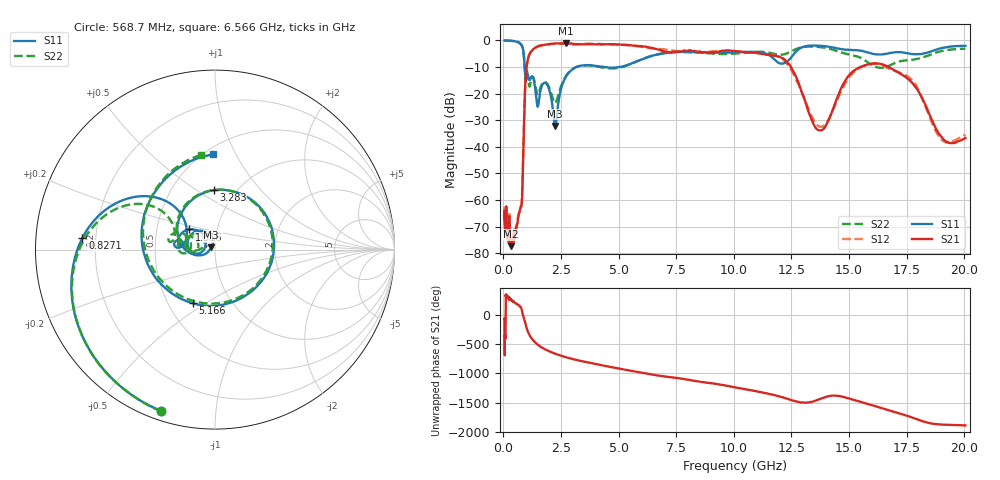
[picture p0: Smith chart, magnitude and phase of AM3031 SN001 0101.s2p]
# Hz S DB R 50
!freq MagS11 AngS11 MagS21 AngS21 MagS12 AngS12 MagS22 AngS22
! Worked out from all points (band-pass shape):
!   1601 points, 50 MHz to 20.05 GHz, reference 50 ohm
!   highest |S21| = -1.06 dB at 2.702 GHz (marker M1); lowest = -77.3 dB at 323 MHz (marker M2)
!   |S21| within 3 dB of the highest: 1.216 GHz to 6.932 GHz (5.716 GHz wide, 140 % of centre); 9.397 GHz to 10.15 GHz (752.8 MHz wide, 7.7 % of centre)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
!   lowest |S11| = -32.2 dB at 2.24 GHz (marker M3), VSWR 1.05, Z = 47.9 + j1.24 ohm
!   |S11| at or under -10 dB: 922 MHz to 3.156 GHz (2.234 GHz wide, 110 % of centre); 4.376 GHz to 5.031 GHz (654.5 MHz wide, 13.9 % of centre)
!   |S22| runs from -23.5 to 0.0 dB; largest |S21 - S12| = 0.067
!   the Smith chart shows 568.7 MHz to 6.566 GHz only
!   S11 on the Smith chart (normalised r, x): 568.7 MHz: 0.04, -0.72; 827.1 MHz: 0.15, +0.04; 1.316 GHz: 0.73, +0.17; 3.283 GHz: 0.79, +0.59; 5.166 GHz: 0.66, -0.44; 6.566 GHz: 0.55, +0.81
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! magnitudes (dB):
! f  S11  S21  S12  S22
! 50 MHz  0.0  -64.8  -64.6  0.0
! 135.9 MHz  0.0  -72.4  -71.9  0.0
! 252.2 MHz  -0.1  -66.5  -65.4  -0.1
! 323 MHz  -0.1  -77.3  -76.4  -0.1
! 369.6 MHz  -0.2  -75.8  -75.6  -0.2
! 568.7 MHz  -0.5  -69.8  -69.6  -0.4
! 827.1 MHz  -2.6  -53.7  -53.6  -2.7
! 1.005 GHz  -13.9  -9.9  -9.8  -11.5
! 1.316 GHz  -14.8  -3.1  -3.2  -14.4
! 1.484 GHz  -24.9  -2.3  -2.2  -20.5
! 1.907 GHz  -16.8  -1.5  -1.6  -16.3
! 2.24 GHz  -32.2  -1.1  -1.2  -23.5
! 2.702 GHz  -13.7  -1.1  -1.3  -13.5
! 2.722 GHz  -13.5  -1.1  -1.3  -13.2
! 3.283 GHz  -9.6  -1.4  -1.4  -9.7
! 5.166 GHz  -9.8  -1.6  -1.6  -10.0
! 6.566 GHz  -5.5  -3.1  -3.1  -5.4
! 7.402 GHz  -4.4  -4.3  -3.9  -4.4
! 11.91 GHz  -8.3  -6.0  -6.0  -5.3
! 13.73 GHz  -2.0  -33.8  -32.4  -2.5
! 16.38 GHz  -5.3  -8.8  -9.2  -10.3
! 20.05 GHz  -2.0  -36.7  -35.5  -3.1
